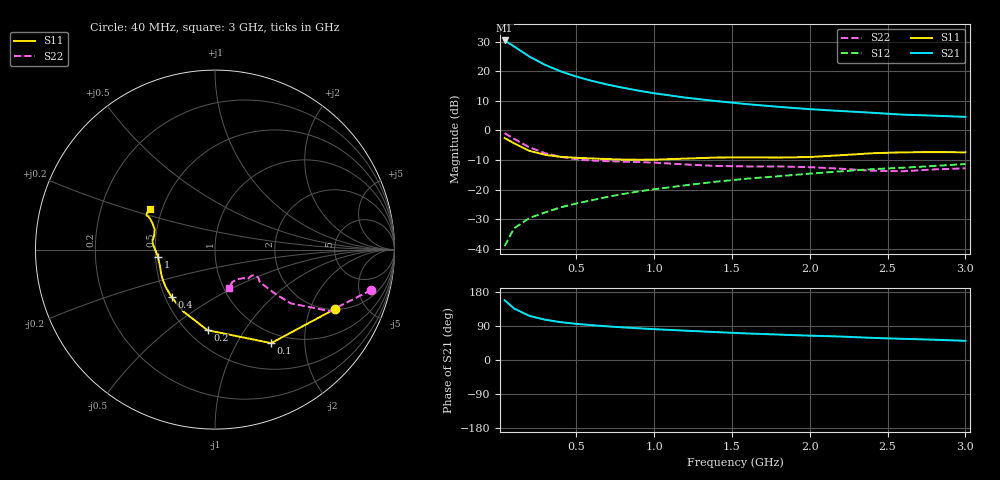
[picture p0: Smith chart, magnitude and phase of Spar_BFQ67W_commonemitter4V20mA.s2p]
! Filename:  BFQ67WE.S2P  Version:  4.0
! NXP part #: BFQ67W  Date: Jun 1994
! Bias condition: Vce=4V, Ic=20mA
#  MHz  S  MA  R  50
! Freq  S11  S21  S12  S22  !GUM [dB]
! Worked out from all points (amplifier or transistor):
!   21 points, 40 MHz to 3 GHz, reference 50 ohm
!   highest |S21| = 30.5 dB at 40 MHz (marker M1)
!   |S21| within 3 dB of that: start of sweep to 128.6 MHz
!   unconditionally stable (mu >= 1): 585.8 MHz to end of sweep
!   at 300 MHz: K = 0.81, MSG = 25.0 dB, |S12| = -27.7 dB
!   at 1 GHz: K = 1.08, MAG = 14.5 dB, |S12| = -19.9 dB
!   at 3 GHz: K = 1.00, MAG = 7.6 dB, |S12| = -11.4 dB
!   lowest NFmin = 2.20 dB at 1 GHz
!   S11 on the Smith chart (normalised r, x): 40 MHz: 2.01, -2.99; 100 MHz: 0.85, -1.40; 200 MHz: 0.62, -0.70; 400 MHz: 0.54, -0.33; 1 GHz: 0.52, -0.05; 3 GHz: 0.43, +0.24
40  0.744 -26.5  33.37 157.8  0.011 77.0  0.9 -14.5
100  0.608 -59.0  26.49 136.1  0.022 65.3  0.725 -28.2
200  0.451 -95.3  17.75 116.3  0.033 60.1  0.517 -35.4
300  0.387 -117.6  12.89 106.3  0.041 61.5  0.413 -36.3
400  0.358 -132.6  10.01 99.9  0.05 63.9  0.357 -36.2
500  0.345 -142.6  8.179 95.4  0.058 65.8  0.326 -36.0
600  0.336 -150.0  6.912 91.9  0.066 67.4  0.31 -35.7
700  0.328 -156.5  5.992 88.8  0.075 69.0  0.302 -35.2
800  0.321 -162.1  5.283 86.1  0.084 69.9  0.297 -34.4
900  0.319 -167.5  4.728 83.7  0.093 70.8  0.292 -33.4
1000  0.32 -172.5  4.269 81.4  0.101 71.3  0.285 -32.7
1200  0.334 179.7  3.601 77.4  0.118 72.2  0.266 -32.6
1400  0.348 174.9  3.145 73.6  0.136 72.9  0.251 -35.1
1600  0.351 171.3  2.786 70.0  0.153 72.4  0.246 -39.4
1800  0.348 167.0  2.51 67.1  0.168 72.7  0.246 -42.0
2000  0.355 161.3  2.294 64.2  0.186 72.9  0.239 -42.9
2200  0.381 156.7  2.134 61.9  0.203 73.2  0.225 -44.9
2400  0.411 153.7  1.995 58.4  0.221 72.8  0.208 -52.2
2600  0.427 153.4  1.849 55.9  0.234 72.0  0.204 -61.7
2800  0.43 152.0  1.78 53.5  0.251 72.2  0.219 -67.2
3000  0.427 148.1  1.698 50.6  0.27 71.7  0.229 -69.6
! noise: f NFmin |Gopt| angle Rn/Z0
1000  2.2  0.82  117  0.245
